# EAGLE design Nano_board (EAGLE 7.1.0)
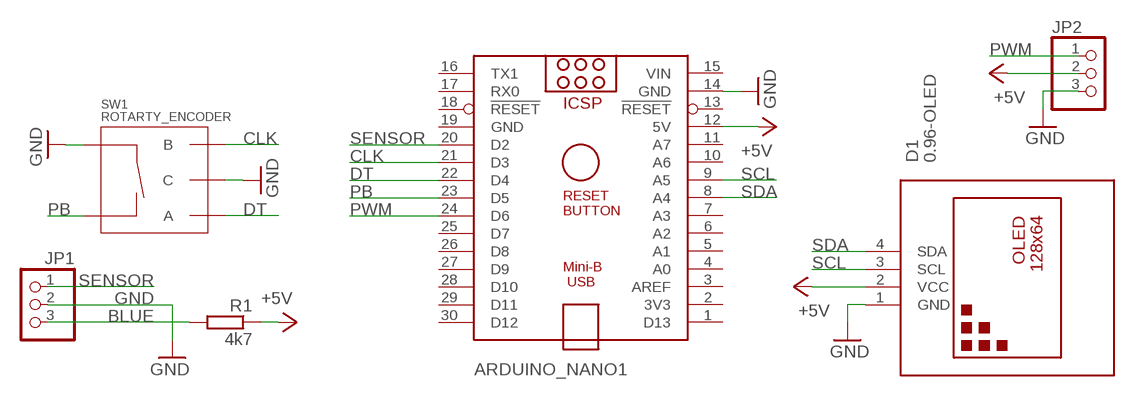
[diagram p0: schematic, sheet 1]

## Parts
ARDUINO_NANO1  ARDUINO_NANO  [ARDUINO_NANO]
D1  0.96-OLED  DISPLAY-OLED-128X64-I2C  [DISPLAY-OLED-128X64-I2C]
JP1  PINHD-1X3/90  [1X03/90]
JP2  PINHD-1X3/90  [1X03/90]
R1  4k7  R-EU_0204/7  [0204/7]
SW1  ROTARTY_ENCODER  [ROTARY_ENC_PLAIN]

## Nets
+5V: ARDUINO_NANO1.12(5V) D1.2(VCC) JP2.2 R1.1
BLUE: JP1.3 R1.2
CLK: ARDUINO_NANO1.21(D3) SW1.B
DT: ARDUINO_NANO1.22(D4) SW1.A
GND: ARDUINO_NANO1.14(GND) D1.1(GND) JP1.2 JP2.3 SW1.C SW1.SW+
PB: ARDUINO_NANO1.23(D5) SW1.SW-
PWM: ARDUINO_NANO1.24(D6) JP2.1
SCL: ARDUINO_NANO1.9(A5) D1.3(SCL)
SDA: ARDUINO_NANO1.8(A4) D1.4(SDA)
SENSOR: ARDUINO_NANO1.20(D2) JP1.1
Unconnected: ARDUINO_NANO1.1(D13) ARDUINO_NANO1.2(3V3) ARDUINO_NANO1.3(AREF) ARDUINO_NANO1.4(A0) ARDUINO_NANO1.5(A1) ARDUINO_NANO1.6(A2) ARDUINO_NANO1.7(A3) ARDUINO_NANO1.10(A6) ARDUINO_NANO1.11(A7) ARDUINO_NANO1.13(!RESET) ARDUINO_NANO1.16(TX1) ARDUINO_NANO1.17(RX0) ARDUINO_NANO1.18(!RESET) ARDUINO_NANO1.25(D7) ARDUINO_NANO1.26(D8) ARDUINO_NANO1.27(D9) ARDUINO_NANO1.28(D10) ARDUINO_NANO1.29(D11) ARDUINO_NANO1.30(D12)

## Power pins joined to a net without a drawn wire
GND: ARDUINO_NANO1.19(GND)
VIN: ARDUINO_NANO1.15(VIN)

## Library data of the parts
ARDUINO_NANO1 = ArduinoNanoV30:ARDUINO_NANO: Arduino Nano V3.0 Overview: The Arduino Nano is a small, complete, and breadboard-friendly board based on the ATmega328 (Arduino Nano 3.x) or ATmega168 (Arduino Nano 2.x). It has more or less the same functionality of the Arduino Duemilanove, but in a different package. It lacks only a DC power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
D1 = diy-modules:DISPLAY-OLED-128X64-I2C: 128x64 Dot Matrix OLED Module based on SSD1306 chip Variant with I2C interface More details available here: http://www.instructables.com/id/Monochrome-096-i2c-OLED-display-with-arduino-SSD13/ SSD1306 datasheet: https://cdn-shop.adafruit.com/datasheets/SSD1306.pdf Click here to find device on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
JP1 JP2 = pinhead:PINHD-1X3: PIN HEADER
R1 = rcl:R-EU_: RESISTOR, European symbol
SW1 = SparkFun-Electromechanical:ROTARTY_ENCODER: Simple no LED rotary encoder Example: COM-09117

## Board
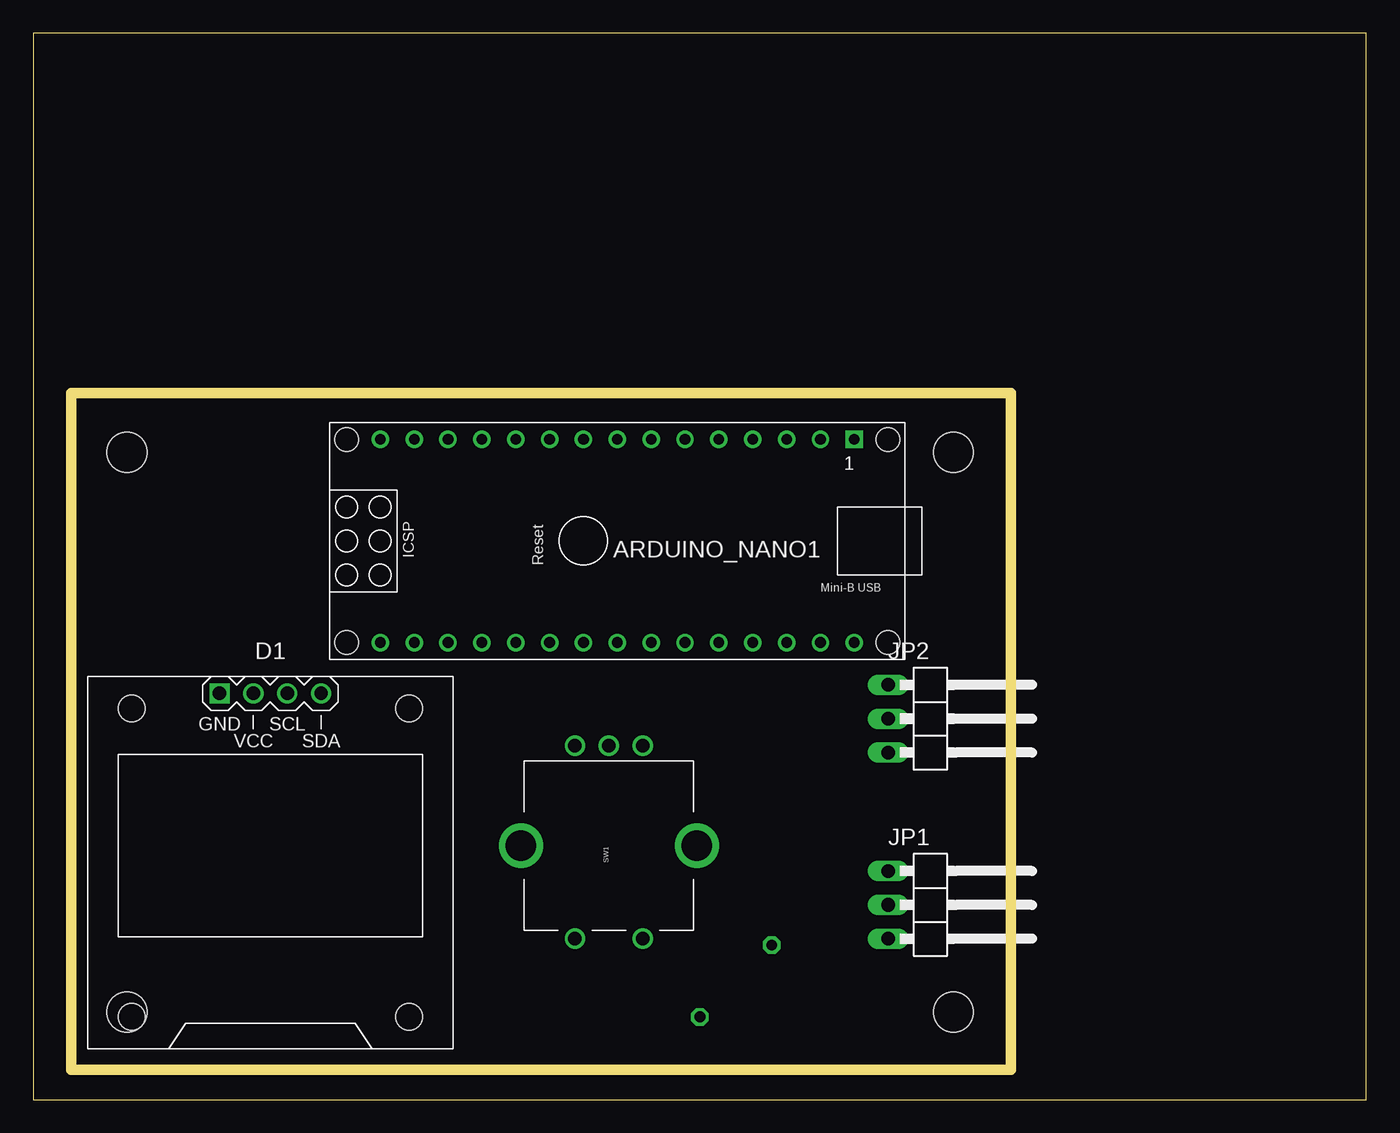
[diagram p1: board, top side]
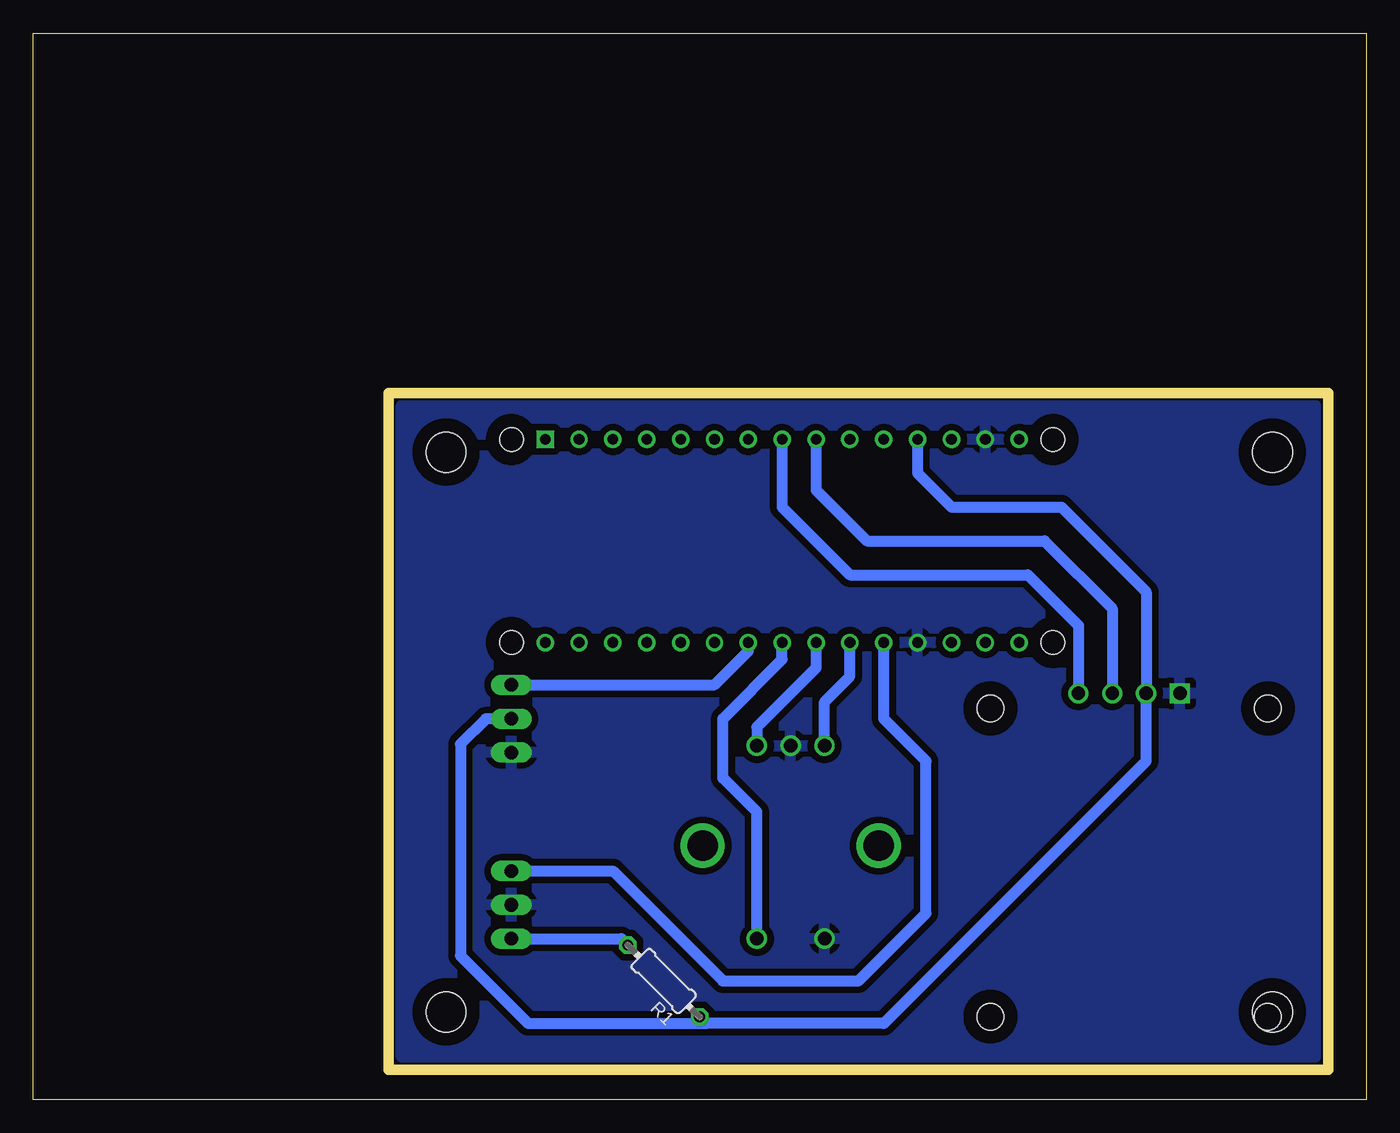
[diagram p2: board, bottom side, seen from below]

Size 100 x 80 mm. Coordinates in mm from the lower left corner, seen from the top.
Outline: 0,0 100,0 100,80 0,80 0,0
Copper layers (1*16): Top 0.035mm / dielectric 1.5mm / Bottom 0.035mm
Design rules "default *": minimum track width 10mil, minimum drill 24mil, track to track 8mil, track to pad 8mil, pad to pad 8mil, via to via 8mil, smd to smd 8mil, copper to edge 40mil, drill to drill 8mil, minimum pad ring 10mil, minimum via ring 8mil, stop-mask expansion 4mil, vias tented up to drill 0mil, thermal gap 18mil
Holes 3 mm at 7.03,48.57 69.03,48.57 69.03,6.57 7.03,6.57
Milling: 4 lines

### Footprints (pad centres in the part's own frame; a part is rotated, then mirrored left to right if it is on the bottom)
ARDUINO_NANO = drill 0.8 square: 1 -20.32,-7.62 | drill 0.8: 2 -17.78,-7.62; 3 -15.24,-7.62; 4 -12.7,-7.62; 5 -10.16,-7.62; 6 -7.62,-7.62; 7 -5.08,-7.62; 8 -2.54,-7.62; 9 0,-7.62; 10 2.54,-7.62; 11 5.08,-7.62; 12 7.62,-7.62; 13 10.16,-7.62; 14 12.7,-7.62; 15 15.24,-7.62; 16 15.24,7.62; 17 12.7,7.62; 18 10.16,7.62; 19 7.62,7.62; 20 5.08,7.62; 21 2.54,7.62; 22 0,7.62; 23 -2.54,7.62; 24 -5.08,7.62; 25 -7.62,7.62; 26 -10.16,7.62; 27 -12.7,7.62; 28 -15.24,7.62; 29 -17.78,7.62; 30 -20.32,7.62 | hole 1.778: -22.86,-7.62; -22.86,7.62; 17.78,7.62; 17.78,-7.62
DISPLAY-OLED-128X64-I2C = drill 1 square: 1 -3.81,12.7 | drill 1: 2 -1.27,12.7; 3 1.27,12.7; 4 3.81,12.7 | hole 2: -10.414,11.557; 10.414,11.557; 10.414,-11.557; -10.414,-11.557
1X03/90 = drill 1.016 long: 1 -2.54,-3.81; 2 0,-3.81; 3 2.54,-3.81
0204/7 = drill 0.813 octagon: 1 -3.81,0; 2 3.81,0
ROTARY_ENC_PLAIN = drill 1.016: A 7.493,-2.54; B 7.493,2.54; C 7.493,0; SW+ -6.985,2.54; SW- -6.985,-2.54 | drill 2.286: P$3 0,6.604; P$4 0,-6.604

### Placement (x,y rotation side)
ARDUINO_NANO1  41.27,41.91 180 top
D1  17.78,17.78 0 top
JP1  67.94,14.61 270 top
JP2  67.94,28.57 270 top
R1  52.7,8.89 135 bottom
SW1  43.18,19.05 90 top

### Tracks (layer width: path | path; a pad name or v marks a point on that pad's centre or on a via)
+5V
  Bottom 0.813: ARDUINO_NANO1.12 33.66,46.99 31.11,44.45 22.86,44.45 16.51,38.1 D1.2 16.51,25.4 36.2,5.71 49.53,5.71 | 49.53,5.71 R1.1 | JP2.2 66.04,28.57 67.94,26.67 67.94,10.79 62.87,5.71 49.53,5.71
BLUE
  Bottom 0.813: JP1.3 55.88,12.06 R1.2
CLK
  Bottom 0.813: SW1.B 40.64,29.84 38.73,31.75 ARDUINO_NANO1.21
DT
  Bottom 0.813: ARDUINO_NANO1.22 41.27,32.38 45.72,27.94 SW1.A
GND
  pour Bottom (isolate 0.508): 3.81,3.17 72.39,3.17 72.39,52.07 3.81,52.07
PB
  Bottom 0.813: SW1.SW- 45.72,21.59 48.26,24.13 48.26,28.57 43.81,33.02 ARDUINO_NANO1.23
PWM
  Bottom 0.813: ARDUINO_NANO1.24 46.35,33.66 48.9,31.11 JP2.1
SCL
  Bottom 0.813: ARDUINO_NANO1.9 41.27,45.72 37.47,41.91 24.13,41.91 19.05,36.83 D1.3
SDA
  Bottom 0.813: ARDUINO_NANO1.8 43.81,44.45 38.73,39.37 25.4,39.37 21.59,35.56 D1.4
SENSOR
  Bottom 0.813: JP1.1 56.52,17.14 48.26,8.89 38.1,8.89 33.02,13.97 33.02,25.4 36.2,28.57 ARDUINO_NANO1.20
